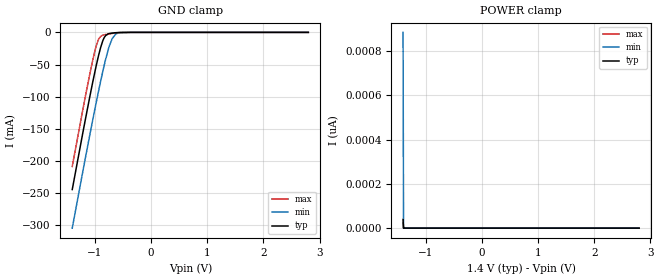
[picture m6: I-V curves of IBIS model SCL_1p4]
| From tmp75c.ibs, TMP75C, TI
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|   Model
[Model]   SCL_1p4
Model_type   Input
Vinl = 0.5
Vinh = 1.3
|   typ   min   max
C_comp   0.318pF   0.315pF   0.322pF
[Voltage Range]   1.4   1.39   1.41
[Temperature Range]   25   125   -40
[Power Clamp Reference]   1.4   1.39   1.41
[GND Clamp Reference]   0   0   0
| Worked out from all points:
|   GND clamp passes 1 mA (typ) near -0.68 V on its own axis
[GND Clamp]
|   Voltage   I(typ)   I(min)   I(max)
-1.4V     -244.5mA   -304.5mA   -208.6mA
-1.161V   -132.8mA   -192.7mA   -96.94mA
-1.035V   -77.01mA   -135.8mA   -42.95mA
-975.8mV  -52.72mA   -110mA     -21.85mA
-929.6mV  -35.17mA   -90.33mA   -10.35mA
-858.2mV  -13.47mA   -61.35mA   -4.432mA
-828.8mV  -7.779mA   -50.16mA   -3.752mA
-744.8mV  -1.867mA   -22.36mA   -2.413mA
-690.2mV  -1.054mA   -9.81mA    -1.678mA
-627.2mV  -535.3uA   -2.661mA   -949.8uA
-350mV    -1.209uA   -5.888uA   -829.8nA
2.8V      0A         0A         0A
[POWER Clamp]
|   Voltage   I(typ)   I(min)   I(max)
-1.4V     39.21pA    885pA      23.3pA
-1.392V   0A         0A         0A
-1.387V   0A         0A         0A
2.8V      0A         0A         0A
